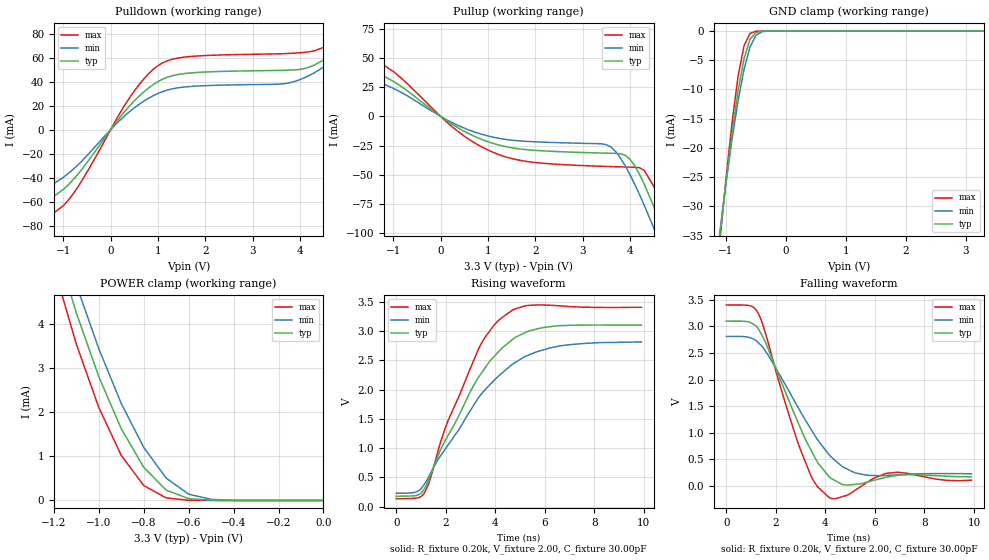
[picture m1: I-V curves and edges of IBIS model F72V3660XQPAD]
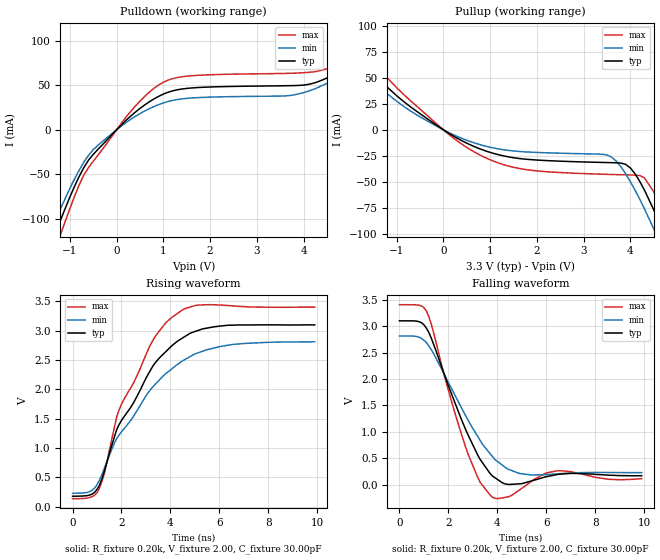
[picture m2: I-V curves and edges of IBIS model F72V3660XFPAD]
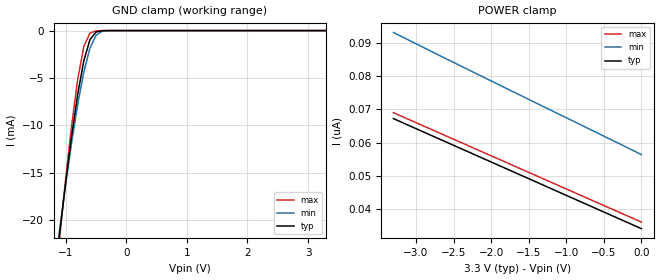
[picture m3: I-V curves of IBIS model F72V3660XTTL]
| IBIS file 72v3660b.ibs created by s2ibis2 version 1.1
| North Carolina State University Electronics Research Laboratory  1995
[IBIS ver]   2.1
[File name]   3660teig.ibs
[File Rev]   1.0
[Date]   08/30/2001
[Source]   Integrated Device Technology, Inc.
[Notes]   1. Temperatures: typ=25C, min=85C, max=-40C 2. Cemos11.5_3v
   process. 3. Ramp rates based on 50 ohm load.
[Copyright]   Copyright 1999, Integrated Device Technology, Inc.
|   Component idt72v3660x
[Component]   idt72v3660x
[Manufacturer]   Integrated Device Technology
[Package]
| variable   typ   min   max
R_pkg   0.75   0.60   0.90
|L_pkg   8.10nH   8.30nH   9.90nH   [jt]
L_pkg   8.30nH   8.10nH   9.90nH   |[jt]
C_pkg   0.53pF   0.46pF   0.60pF
[Pin]  signal_name   model_name   R_pin   L_pin   C_pin
A1   ASYWL   F72V3660XTTL
A2   WENL   F72V3660XTTL
A3   WCLK   F72V3660XTTL
A4   PAFL   F72V3660XFPAD
A5   FFL   F72V3660XFPAD
A6   HFL   F72V3660XFPAD
A7   BML   F72V3660XTTL
A8   EFL   F72V3660XFPAD
A9   RCLK   F72V3660XTTL
A10   RENL   F72V3660XTTL
A11   OEL   F72V3660XTTL
A12   Q35   F72V3660XQPAD
B1   SENL   F72V3660XTTL
B2   IW   F72V3660XTTL
B3   PRSL   F72V3660XTTL
B4   LDL   F72V3660XTTL
B5   MRSL   F72V3660XTTL
B6   FS0   F72V3660XTTL
B7   FS1   F72V3660XTTL
B8   ASYRL   F72V3660XTTL
B9   IP   F72V3660XTTL
B10   PFM   F72V3660XTTL
B11   RTL   F72V3660XTTL
B12   Q34   F72V3660XQPAD
C1   D35   F72V3660XTTL
C2   D34   F72V3660XTTL
C3   D33   F72V3660XTTL
C4   FWFTSI   F72V3660XTTL
C5   OW   F72V3660XTTL
C6   VCC   POWER
C7   VCC   POWER
C8   BEL   F72V3660XTTL
C9   PAEL   F72V3660XFPAD
C10   RM   F72V3660XTTL
C11   Q32   F72V3660XQPAD
C12   Q33   F72V3660XQPAD
D1   D32   F72V3660XTTL
D2   D31   F72V3660XTTL
D3   D30   F72V3660XTTL
D4   VCC   POWER
D5   VCC   POWER
D6   GND   GND
D7   GND   GND
D8   VCC   POWER
D9   VCC   POWER
D10   Q29   F72V3660XQPAD
D11   Q30   F72V3660XQPAD
D12   Q31   F72V3660XQPAD
E1   D29   F72V3660XTTL
E2   D28   F72V3660XTTL
E3   D27   F72V3660XTTL
E4   VCC   POWER
E5   GND   GND
E6   GND   GND
E7   GND   GND
E8   GND   GND
E9   VCC   POWER
E10   Q26   F72V3660XQPAD
E11   Q27   F72V3660XQPAD
E12   Q28   F72V3660XQPAD
F1   D26   F72V3660XTTL
F2   D25   F72V3660XTTL
F3   D24   F72V3660XTTL
F4   VCC   POWER
F5   GND   GND
F6   GND   GND
F7   GND   GND
F8   GND   GND
F9   VCC   POWER
F10   Q23   F72V3660XQPAD
F11   Q24   F72V3660XQPAD
F12   Q25   F72V3660XQPAD
G1   D21   F72V3660XTTL
G2   D22   F72V3660XTTL
G3   D23   F72V3660XTTL
G4   VCC   POWER
G5   GND   GND
G6   GND   GND
G7   GND   GND
G8   GND   GND
G9   VCC   POWER
G10   Q22   F72V3660XQPAD
G11   Q21   F72V3660XQPAD
G12   Q20   F72V3660XQPAD
H1   D18   F72V3660XTTL
H2   D19   F72V3660XTTL
H3   D20   F72V3660XTTL
H4   VCC   POWER
H5   GND   GND
H6   GND   GND
H7   GND   GND
H8   GND   GND
H9   VCC   POWER
H10   Q19   F72V3660XQPAD
H11   Q18   F72V3660XQPAD
H12   Q17   F72V3660XQPAD
J1   D15   F72V3660XTTL
J2   D16   F72V3660XTTL
J3   D17   F72V3660XTTL
J4   VCC   POWER
J5   VCC   POWER
J6   GND   GND
J7   GND   GND
J8   VCC   POWER
J9   VCC   POWER
J10   Q16   F72V3660XQPAD
J11   Q15   F72V3660XQPAD
J12   Q14   F72V3660XQPAD
K1   D12   F72V3660XTTL
K2   D13   F72V3660XTTL
K3   D14   F72V3660XTTL
K4   D3   F72V3660XTTL
K5   D0   F72V3660XTTL
K6   VCC   POWER
K7   VCC   POWER
K8   NC   NC
K9   Q2   F72V3660XQPAD
K10   Q13   F72V3660XQPAD
K11   Q12   F72V3660XQPAD
K12   Q11   F72V3660XQPAD
L1   D10   F72V3660XTTL
L2   D11   F72V3660XTTL
L3   D6   F72V3660XTTL
L4   D4   F72V3660XTTL
L5   D1   F72V3660XTTL
L6   NC   NC
L7   NC   NC
L8   Q0   F72V3660XQPAD
L9   Q3   F72V3660XQPAD
L10   Q5   F72V3660XQPAD
L11   Q10   F72V3660XQPAD
L12   Q9   F72V3660XQPAD
M1   D9   F72V3660XTTL
M2   D8   F72V3660XTTL
M3   D7   F72V3660XTTL
M4   D5   F72V3660XTTL
M5   D2   F72V3660XTTL
M6   NC   NC
M7   NC   NC
M8   Q1   F72V3660XQPAD
M9   Q4   F72V3660XQPAD
M10   Q6   F72V3660XQPAD
M11   Q7   F72V3660XQPAD
M12   Q8   F72V3660XQPAD
| Models and submodels in the file (3): F72V3660XQPAD (3-state), F72V3660XFPAD (Output), F72V3660XTTL (Input)
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| FIN  FIN   dummy_model
| QIN  QIN   dummy_model
| QOEL QOEL   dummy_model
|   Model F72V3660XQPAD
[Model]   F72V3660XQPAD
Model_type   3-state
Polarity   Non-Inverting
Enable   Active-Low
|Vinl =  0.000V   [jt]
|Vinh =  3.000V   [jt]
Vmeas =  1.500V
C_comp   3.00pF   NA   NA
[Temperature Range]   25.00   85.00   -40.00
[Voltage Range]   3.30V   3.00V   3.60V
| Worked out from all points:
|   slope of the pulldown table from 0 to 0.495 V, typ, clamps not added: 20.9 ohm
|   slope of the pullup table from 0 to 0.495 V, typ, clamps not added: 39 ohm
|   GND clamp passes 1 mA (typ) near -0.57 V on its own axis
|   POWER clamp passes 1 mA (typ) near -0.83 V on its own axis
|   rising waveform, R_fixture 0.20k, V_fixture 2.00, C_fixture 30.00pF: 20-80 % time 2.26ns typ, 2.7ns min, 1.81ns max; typ from 0.179 V to 3.1 V
|   falling waveform, R_fixture 0.20k, V_fixture 2.00, C_fixture 30.00pF: 20-80 % time 1.58ns typ, 1.99ns min, 1.27ns max; typ from 3.1 V to 0.172 V
[Pulldown]
| voltage   I(typ)   I(min)   I(max)
-3.3V     -78.1mA    -69.1mA    -88.4mA
-1.9V     -70.5mA    -59.2mA    -83.7mA
-1.5V     -64.03mA   -52.53mA   -78.38mA
-1V       -49.8mA    -39.74mA   -63.32mA
-600mV    -32.63mA   -25.8mA    -41.94mA
400mV     19.75mA    15.01mA    26.5mA
1.1V      42.09mA    31.72mA    55.68mA
3.8V      49.61mA    39.21mA    63.53mA
4.5V      58.01mA    52.1mA     68.44mA
4.9V      71.41mA    65.07mA    81.85mA
5.3V      92.34mA    83.36mA    107mA
6.6V      239mA      203mA      293mA
[Pullup]
| voltage   I(typ)   I(min)   I(max)
-3.3V     63.83mA    53.96mA    75.83mA
-1.5V     40.98mA    32.98mA    51.93mA
300mV     -8.18mA    -6.429mA   -10.76mA
1.1V      -22.96mA   -17.67mA   -30.55mA
1.9V      -28.69mA   -21.5mA    -38.93mA
3.5V      -31.4mA    -24.13mA   -42.74mA
4V        -36.59mA   -49.74mA   -43.32mA
4.3V      -57.78mA   -75.78mA   -46.12mA
4.5V      -76.76mA   -95.06mA   -59.46mA
4.7V      -97.6mA    -115mA     -79.6mA
4.9V      -119mA     -136mA     -102mA
6.6V      -313mA     -320mA     -309mA
[GND_clamp]
| voltage   I(typ)   I(min)   I(max)
-3.3V     -278mA     -262mA     -298mA
-1.1V     -34.79mA   -34.08mA   -35.63mA
-1V       -25.68mA   -25.97mA   -25.14mA
-900mV    -17.4mA    -18.54mA   -15.66mA
-800mV    -10.26mA   -11.98mA   -7.802mA
-700mV    -4.731mA   -6.568mA   -2.51mA
-600mV    -1.413mA   -2.718mA   -390uA
-500mV    -228uA     -719uA     -31.26uA
-400mV    -22.15uA   -115uA     -1.32uA
-300mV    -1.402uA   -12.89uA   -32.97nA
3.3V      34.83nA    488nA      33.01nA
[POWER_clamp]
| voltage   I(typ)   I(min)   I(max)
-3.3V     72.27mA    66.54mA    80.97mA
-1.2V     5.92mA     6.51mA     5.285mA
-1.1V     4.244mA    4.879mA    3.539mA
-1V       2.802mA    3.433mA    2.105mA
-900mV    1.623mA    2.194mA    1.02mA
-800mV    751uA      1.201mA    338uA
-700mV    234uA      506uA      58.4uA
-600mV    41.73uA    142uA      5.351uA
-500mV    4.842uA    25.8uA     348nA
-400mV    454nA      3.649uA    51.06nA
0V        34.83nA    78.19nA    36.01nA
[Ramp]
| variable   typ   min   max
dV/dt_r   0.86/0.74n   0.65/0.97n   1.13/0.58n
dV/dt_f   1.29/0.94n   1.02/1.24n   1.58/0.64n
R_load = 50.00
[Rising Waveform]
R_fixture = 0.20k
V_fixture = 2.00
C_fixture = 30.00pF
R_dut = 0.75
L_dut = 8.10nH
C_dut = 0.53pF
| time   V(typ)   V(min)   V(max)
0s        179mV      229mV      137mV
800ps     191mV      250mV      146mV
1.1ns     281mV      361mV      211mV
1.3ns     446mV      500mV      381mV
2ns       1.146V     996mV      1.368V
3.3ns     2.193V     1.848V     2.668V
4.2ns     2.677V     2.256V     3.205V
5.2ns     2.973V     2.564V     3.43V
6.2ns     3.073V     2.71V      3.439V
9.9ns     3.1V       2.812V     3.404V
[Falling Waveform]
R_fixture = 0.20k
V_fixture = 2.00
C_fixture = 30.00pF
R_dut = 0.75
L_dut = 8.10nH
C_dut = 0.53pF
| time   V(typ)   V(min)   V(max)
0s        3.1V       2.813V     3.405V
1ns       3.071V     2.783V     3.384V
1.3ns     2.949V     2.691V     3.236V
1.8ns     2.45V      2.375V     2.505V
3ns       1.083V     1.394V     676mV
3.5ns     603mV      1.006V     116mV
4.2ns     150mV      560mV      -231mV
5.2ns     30.62mV    247mV      -80.64mV
6.5ns     169mV      199mV      239mV
9.9ns     172mV      230mV      109mV
|   Model F72V3660XFPAD
[Model]   F72V3660XFPAD
Model_type   Output
Polarity   Non-Inverting
Enable   Active-Low
|Vinl =  0.000V   [jt]
|Vinh =  3.000V   [jt]
Vmeas =  1.500V
C_comp   3.00pF   NA   NA
[Temperature Range]   25.00   85.00   -40.00
[Voltage Range]   3.30V   3.00V   3.60V
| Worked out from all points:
|   slope of the pulldown table from 0 to 0.495 V, typ, clamps not added: 20.9 ohm
|   slope of the pullup table from 0 to 0.495 V, typ, clamps not added: 39 ohm
|   rising waveform, R_fixture 0.20k, V_fixture 2.00, C_fixture 30.00pF: 20-80 % time 2.1ns typ, 2.51ns min, 1.75ns max; typ from 0.179 V to 3.1 V
|   falling waveform, R_fixture 0.20k, V_fixture 2.00, C_fixture 30.00pF: 20-80 % time 1.49ns typ, 1.82ns min, 1.2ns max; typ from 3.1 V to 0.172 V
[Pulldown]
| voltage   I(typ)   I(min)   I(max)
-3.3V     -2.813A    -331mA     -386mA
-1.5V     -140mA     -123mA     -161mA
-1V       -75.48mA   -65.71mA   -88.46mA
-700mV    -42.28mA   -36.27mA   -50.74mA
-500mV    -27.61mA   -22.34mA   -35.37mA
400mV     19.75mA    15.01mA    26.5mA
1.1V      42.09mA    31.72mA    55.68mA
4V        50.16mA    41.67mA    64.04mA
4.9V      71.41mA    65.07mA    81.85mA
5.3V      92.34mA    83.36mA    107mA
5.7V      123mA      109mA      145mA
6.6V      239mA      203mA      293mA
[Pullup]
| voltage   I(typ)   I(min)   I(max)
-3.3V     136mA      120mA      157mA
-2.5V     97.91mA    85.33mA    115mA
-2.1V     79.57mA    68.81mA    94.27mA
-700mV    21.96mA    17.97mA    27.81mA
900mV     -20.19mA   -15.64mA   -26.76mA
3.5V      -31.4mA    -24.13mA   -42.74mA
4V        -36.59mA   -49.74mA   -43.32mA
4.3V      -57.78mA   -75.78mA   -46.12mA
4.5V      -76.76mA   -95.06mA   -59.46mA
4.7V      -97.6mA    -115mA     -79.6mA
4.9V      -119mA     -136mA     -102mA
6.6V      -313mA     -320mA     -309mA
[Ramp]
| variable   typ   min   max
dV/dt_r   0.86/0.44n   0.65/0.52n   1.13/0.39n
dV/dt_f   1.29/0.69n   1.02/0.88n   1.58/0.51n
R_load = 50.00
[Rising Waveform]
R_fixture = 0.20k
V_fixture = 2.00
C_fixture = 30.00pF
R_dut = 0.75
L_dut = 8.10nH
C_dut = 0.53pF
| time   V(typ)   V(min)   V(max)
0s        179mV      229mV      137mV
1ns       297mV      375mV      239mV
1.3ns     609mV      657mV      565mV
1.8ns     1.31V      1.159V     1.524V
2ns       1.471V     1.278V     1.749V
3.3ns     2.41V      2.052V     2.849V
4.1ns     2.76V      2.365V     3.242V
5ns       2.988V     2.606V     3.431V
6ns       3.079V     2.729V     3.44V
9.9ns     3.1V       2.813V     3.404V
[Falling Waveform]
R_fixture = 0.20k
V_fixture = 2.00
C_fixture = 30.00pF
R_dut = 0.75
L_dut = 8.10nH
C_dut = 0.53pF
| time   V(typ)   V(min)   V(max)
0s        3.1V       2.813V     3.405V
800ps     3.084V     2.79V      3.394V
1.1ns     2.961V     2.688V     3.286V
2.8ns     948mV      1.226V     586mV
3.3ns     480mV      839mV      46.94mV
3.8ns     167mV      536mV      -235mV
4.3ns     19.09mV    338mV      -238mV
4.9ns     19.4mV     215mV      -100mV
6.5ns     199mV      209mV      268mV
9.9ns     172mV      230mV      117mV
|   Model F72V3660XTTL
[Model]   F72V3660XTTL
Model_type   Input
|Vinl =  0.000V   [jt]
|Vinh =  3.000V   [jt]
Vinl =  0.800V   | [jt]
Vinh =  2.000V   | [jt]
|Vmeas =  1.500V   [jt]
C_comp   3.00pF   NA   NA
|[Temperature Range]   25.00   85.00   -40.00
|[Voltage Range]   3.30V   3.00V   3.60V
|[GND_clamp]
[Temperature Range]   25.00   85.00   -40.00
[Pullup Reference]   3.30V   3.00V   3.60V
[Pulldown Reference]   0.000V   0.000V   0.000V
[POWER Clamp Reference]   3.30V   3.00V   3.60V
[GND Clamp Reference]   0.000V   0.000V   0.000V
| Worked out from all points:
|   GND clamp passes 1 mA (typ) near -0.60 V on its own axis
[GND_clamp]
| voltage   I(typ)   I(min)   I(max)
-3.3V     -163mA     -152mA     -175mA
-1.2V     -27.14mA   -26.04mA   -28.44mA
-1.1V     -21.44mA   -20.99mA   -21.88mA
-1V       -16.05mA   -16.21mA   -15.65mA
-900mV    -11.07mA   -11.76mA   -9.94mA
-800mV    -6.681mA   -7.76mA    -5.083mA
-700mV    -3.176mA   -4.372mA   -1.687mA
-600mV    -978uA     -1.868mA   -273uA
-500mV    -164uA     -509uA     -22.75uA
-400mV    -16.27uA   -84.16uA   -951nA
-300mV    -1.023uA   -9.558uA   -24.55nA
3.3V      34.02nA    59.73nA    33.01nA
[POWER_clamp]
| voltage   I(typ)   I(min)   I(max)
-3.3V     67.23nA    93.23nA    69.01nA
-2.9V     63.2nA     88.67nA    65.01nA
-2.3V     57.16nA    81.94nA    59.01nA
0V        34.02nA    56.39nA    36.01nA
